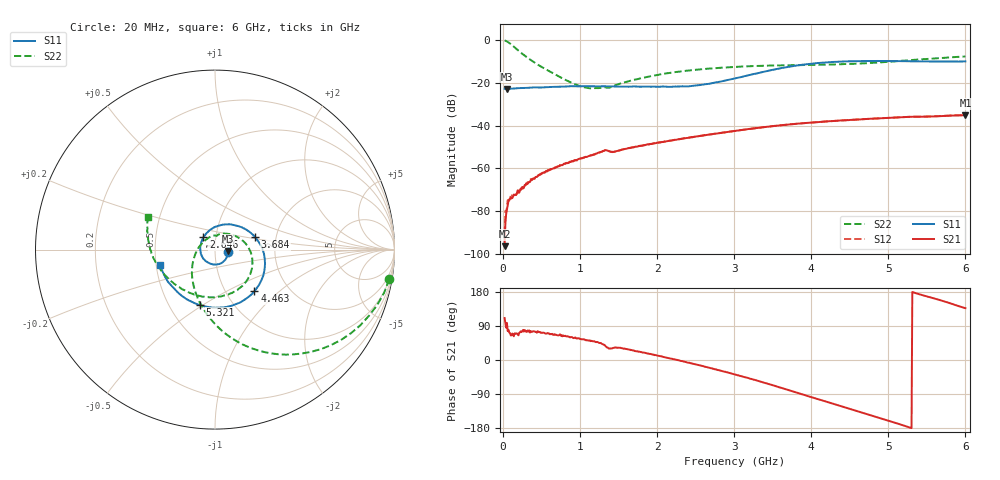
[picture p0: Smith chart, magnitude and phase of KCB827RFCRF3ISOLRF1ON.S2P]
!Agilent Technologies,E5071B,JP1KK00126,A.08.11
!Date: Tue May 06 07:22:48 2014
!Data & Calibration Information:
!Freq	S11:SOLT2(ON)	S21:SOLT2(ON)	S12:SOLT2(ON)	S22:SOLT2(ON)
# Hz S dB R 50
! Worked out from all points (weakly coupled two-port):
!   600 points, 20 MHz to 6 GHz, reference 50 ohm
!   highest |S21| = -35.11 dB at 6 GHz (marker M1); lowest = -96.4 dB at 20 MHz (marker M2)
!   lowest |S11| = -22.8 dB at 49.95 MHz (marker M3), VSWR 1.16, Z = 57.7 - j0.903 ohm
!   |S11| at or under -10 dB: start of sweep to 4.408 GHz; 5.646 GHz to 5.776 GHz (130.2 MHz wide, 2.28 % of centre); 5.906346 GHz to 5.913075 GHz (6.729 MHz wide, 0.114 % of centre)
!   |S22| runs from -22.6 to -0.1 dB; largest |S21 - S12| = 0.00015
!   S11 on the Smith chart (normalised r, x): 20 MHz: 1.15, -0.03; 2.646 GHz: 0.87, +0.12; 3.684 GHz: 1.55, +0.23; 4.463 GHz: 1.36, -0.70; 5.321 GHz: 0.71, -0.49; 6 GHz: 0.52, -0.10
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2e7  -22.73 -11.5  -96.40 110.7  -90.49 -31.9  -0.13 -9.6
4.994992e7  -22.84 -6.2  -79.25 97.9  -78.47 82.9  -0.60 -23.3
8.988314e7  -22.76 -6.8  -74.14 70.9  -73.29 70.1  -1.54 -39.4
1.397997e8  -22.62 -9.0  -72.23 62.6  -72.62 62.9  -3.04 -56.1
2.196661e8  -22.40 -13.3  -70.41 73.0  -69.88 75.1  -5.50 -75.9
3.294825e8  -22.27 -21.9  -66.59 74.9  -66.42 74.6  -8.55 -95.5
5.690818e8  -22.05 -39.0  -61.48 70.0  -61.29 71.0  -13.93 -129.2
1.018331e9  -21.54 -72.8  -55.23 54.6  -55.30 56.3  -21.77 157.0
1.31783e9  -21.56 -96.6  -51.56 39.8  -51.59 39.9  -22.03 90.4
1.37773e9  -21.65 -101.8  -51.98 29.8  -51.92 30.4  -22.24 83.1
1.447613e9  -21.68 -107.8  -52.27 32.5  -52.12 32.1  -21.21 76.5
2.016661e9  -21.79 -157.7  -47.89 11.0  -47.97 11.6  -16.19 21.7
2.645609e9  -20.51 132.8  -44.28 -18.7  -44.29 -19.3  -13.39 -14.1
3.014992e9  -17.85 88.0  -42.46 -38.3  -42.44 -38.2  -12.49 -33.2
3.364407e9  -14.95 48.7  -40.81 -58.3  -40.80 -58.5  -12.00 -50.9
3.683873e9  -12.64 17.2  -39.55 -78.0  -39.51 -78.4  -11.73 -68.1
4.013322e9  -10.94 -11.6  -38.51 -98.8  -38.50 -98.9  -11.58 -87.6
4.462571e9  -9.91 -46.5  -37.43 -126.7  -37.41 -127.1  -11.17 -116.5
5.011653e9  -9.77 -83.6  -36.33 -160.8  -36.31 -161.1  -10.08 -153.2
5.321135e9  -9.89 -105.3  -35.84 178.8  -35.82 178.6  -9.21 -172.0
5.630618e9  -9.99 -130.1  -35.62 160.5  -35.61 160.3  -8.47 171.3
6e9  -9.93 -164.4  -35.11 136.8  -35.09 136.6  -7.64 153.7
